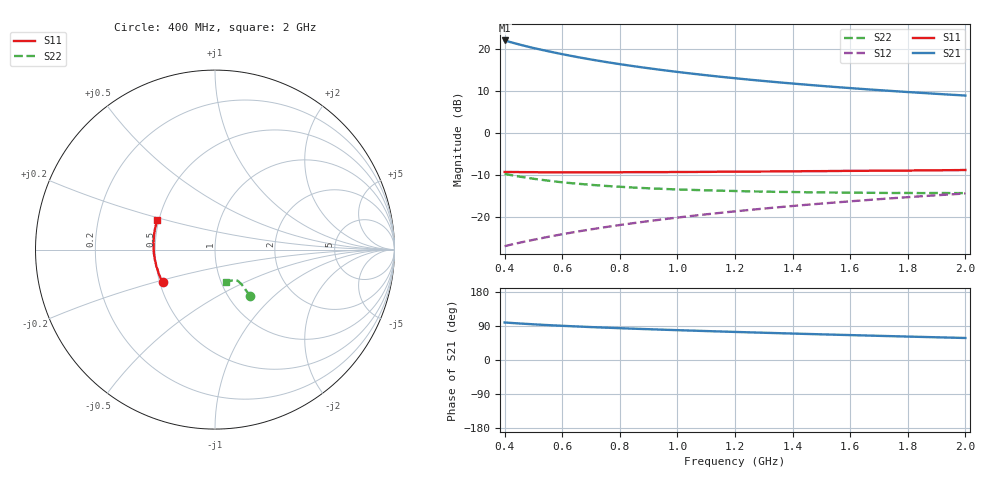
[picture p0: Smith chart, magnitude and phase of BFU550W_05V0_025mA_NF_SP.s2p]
! Filename:  P:\Prog\Test\Noise\ATS_data\Testdata_Net\06 Compressed Noise after Statistics\BFU550W_APM2013_11_D05_05p0V_025mA_NF_CM01_D.sf
! Date/Time: Tue 26/Mar/2013 16:25:23
! BFU550W_APM2013_11_D05_05p0V_1to35mA_NF_CM01_Bias8_R.sf
! Noise Parameter Data File
! BFU550W_APM2013_11_D05_05p0V_1to35mA_NF_CM01
! Date/time: Mon Mar 25 13:26:50 2013
! VAR V_out= 5.000000
! VAR I_out= 25.005000
! VAR V_in= 0.825500
! VAR I_in= 0.263500
! Device data file deembeded for feedlines and parallel
! Original file: \06 Compressed Noise after Statistics\BFU550W_APM2013_11_D05_05p0V_025mA_NF_CM01_R.sf
! Feed-files: PR019V01_070313_Feed1.s2p, PR019V01_070313_Feed2.s2p
! Parallel-file: PR019V01_070313_Par.s2p
# MHz S MA R 50
!  Freq-MHz  S11-mag  S11-arg  S21-mag  S21-arg  S12-mag  S12-arg  S22-mag  S22-arg
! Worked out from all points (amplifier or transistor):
!   37 points, 400 MHz to 2 GHz, reference 50 ohm
!   highest |S21| = 22.0 dB at 400 MHz (marker M1)
!   |S21| within 3 dB of that: start of sweep to 581.3 MHz
!   unconditionally stable (mu >= 1): 958.5 MHz to end of sweep
!   at 500 MHz: K = 0.92, MSG = 22.8 dB, |S12| = -25.5 dB
!   at 1.1 GHz: K = 1.01, MAG = 16.1 dB, |S12| = -19.4 dB
!   at 2 GHz: K = 1.00, MAG = 11.3 dB, |S12| = -14.4 dB
!   lowest NFmin = 1.03 dB at 480 MHz
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400  0.3428 -148.1  12.63 99.0  0.04478 68.0  0.3251 -52.7
420  0.3423 -150.2  12.08 97.9  0.04651 68.3  0.3158 -52.7
440  0.342 -152.1  11.57 96.9  0.0482 68.5  0.3067 -52.7
460  0.3415 -153.8  11.11 96.0  0.04992 68.8  0.2988 -52.8
480  0.341 -155.5  10.68 95.1  0.05164 69.1  0.2917 -52.8
500  0.341 -157.2  10.28 94.2  0.05332 69.3  0.2847 -52.7
550  0.3385 -160.7  9.416 92.1  0.05773 69.9  0.2704 -52.7
600  0.3398 -163.9  8.674 90.2  0.06214 70.3  0.258 -52.6
650  0.339 -166.8  8.04 88.5  0.06657 70.6  0.249 -52.6
700  0.3393 -169.4  7.491 86.9  0.07103 70.9  0.2408 -52.8
750  0.3399 -171.7  7.015 85.4  0.07549 71.0  0.2339 -52.9
800  0.3399 -174.1  6.596 84.0  0.08 71.2  0.2286 -53.3
850  0.3411 -176.2  6.225 82.6  0.08446 71.2  0.2231 -53.3
950  0.3412 -179.8  5.598 80.0  0.09358 71.3  0.2154 -54.0
1050  0.3429 176.8  5.089 77.5  0.1027 71.1  0.2097 -55.0
1150  0.3452 173.5  4.665 75.2  0.1118 70.9  0.205 -56.1
1200  0.3451 172.1  4.484 74.1  0.1164 70.7  0.2033 -56.9
1350  0.3478 168.0  4.011 70.8  0.1302 70.1  0.1985 -58.8
1500  0.3506 164.1  3.633 67.7  0.144 69.3  0.1961 -61.4
1650  0.3539 160.4  3.324 64.7  0.1578 68.4  0.1939 -64.0
1750  0.3559 158.4  3.151 62.8  0.1671 67.8  0.1925 -65.9
2000  0.3617 152.9  2.789 58.1  0.1901 66.0  0.1919 -71.4
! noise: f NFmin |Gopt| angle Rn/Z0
400  1.04  0.3365  -173.8  0.0668
460  1.048  0.3392  -172.1  0.0659
600  1.046  0.3508  -169.2  0.0682
800  1.093  0.3716  -164.8  0.0637
1000  1.121  0.3764  -160.8  0.0675
1200  1.159  0.3907  -156  0.0697
1400  1.218  0.3984  -152.9  0.0707
1600  1.234  0.3788  -149.3  0.0864
1800  1.239  0.4135  -144.4  0.0907
2000  1.256  0.4214  -140.3  0.1002
